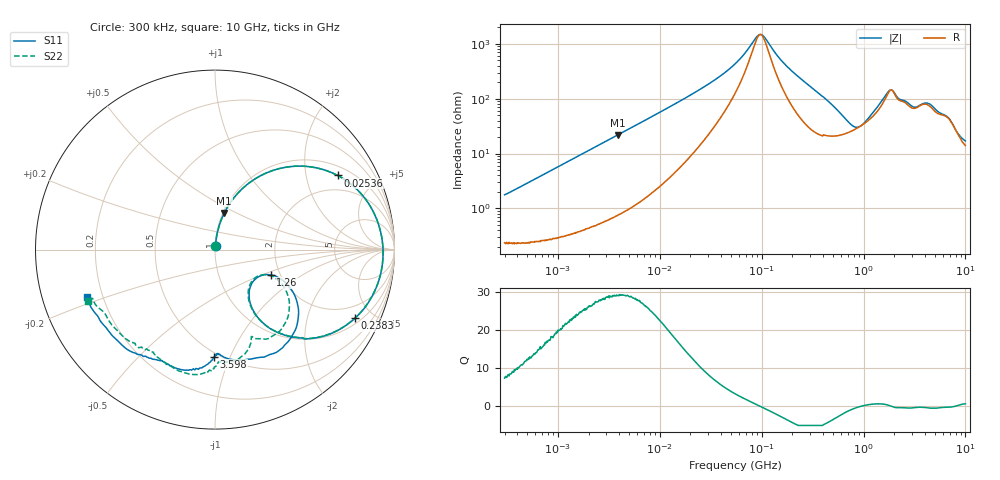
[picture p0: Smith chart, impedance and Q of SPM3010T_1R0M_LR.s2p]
! S-Parameter Data Generated by TDK Corporation
! Copyright(C) 2019 TDK Corporation.
! All Rights Reserved.
! TDK P/N: SPM3010T-1R0M-LR (Inductor)
! Property: L=1uH at 100kHz
! Size(LxWxT): 3.2x3x1mm
! Model Type: s2p (Touchstone File Format Version 1.0)
! Frequency: DC=Yes Start=0.3MHz Stop=10000MHz 802points Log-sweep
! Model Generated on Sep. 23, 2019
! Port Assignments:
!  1 ---@@@--- 2
! Applicable Conditions:
!  Temperature = 25 degC
!  DC Bias Current = 0 A
!  Small Signal Operation
! Terms and conditions regarding TDK Simulation Models
! (1)This simulation model is being provided solely for informational purposes. Please refer to the specifications of the products in terms of detailed characteristics of such products.
! (2)In no event shall TDK Corporation of any of its subsidiaries be liable for any loss or damage arising, directly or indirectly,
!  From any information contained in this simulation model, including, but not limited to loss or damages arising from any inaccuracies, omissions or errors in connection with such information.
! (3)Any and all copyrights on this simulation model are owned by TDK Corporation.
!  Duplication or redistribution of this simulation model without prior written permission from TDK Corporation is prohibited.
! (4)This simulation model is subject to any modification or change without any prior notice.
! (5)Neither TDK Corporation nor any of its subsidiaries shall make any warranty, express or implied,
!  Including but not limited to the correctness, implied warranties of merchantability and fitness for a particular purpose with respect to this simulation models.
! (6)The use of this simulation model shall be deemed to have consented to the terms and conditions hereof.
# Hz S MA R 50
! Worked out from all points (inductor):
!   801 points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, 300 kHz to 10 GHz, reference 50 ohm
!   read as one part in series: L = 916 nH near 318.3 kHz
!   highest Q = 29.1 at 3.867 MHz (marker M1), where L = 896 nH
!   self-resonance near 97.29 MHz
!   S11 on the Smith chart (normalised r, x): 300 kHz: 1.00, +0.04; 25.36 MHz: 1.34, +3.05; 238.3 MHz: 1.26, -3.94; 1.26 GHz: 1.79, -0.57; 3.598 GHz: 0.47, -0.87; 10 GHz: 0.14, -0.18
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300000  0.01837 81.3  0.9974 -1.0  0.9976 -0.9  0.0181 82.0
1713600  0.0964 82.1  0.9913 -5.5  0.9916 -5.5  0.09641 82.2
3866967  0.2107 75.8  0.9701 -12.2  0.9705 -12.2  0.2108 75.8
9671944  0.4691 59.3  0.8626 -28.1  0.8632 -28.1  0.469 59.3
2.53611e7  0.7983 31.2  0.5288 -53.2  0.5291 -53.2  0.7982 31.2
5.477226e7  0.9168 10.6  0.2138 -62.6  0.2139 -62.6  0.9167 10.6
9.914192e7  0.937 -2.6  0.06343 3.4  0.06346 3.4  0.9368 -2.6
1.473106e8  0.9261 -12.0  0.1629 55.5  0.163 55.4  0.9258 -11.9
2.382595e8  0.8692 -26.1  0.359 53.2  0.3591 53.2  0.8683 -26.1
3.126428e8  0.7984 -35.8  0.4859 44.8  0.4862 44.8  0.797 -35.9
4.687561e8  0.6178 -50.7  0.658 26.5  0.6583 26.5  0.615 -50.6
6.987102e8  0.3875 -57.7  0.7528 4.2  0.7532 4.1  0.382 -58.0
9.67469e8  0.277 -40.8  0.7342 -15.3  0.7345 -15.3  0.2704 -40.8
1.260284e9  0.3417 -24.4  0.6452 -31.6  0.6454 -31.6  0.3374 -25.3
1.525386e9  0.4646 -26.7  0.5179 -42.4  0.5181 -42.4  0.4567 -30.0
1.767019e9  0.5914 -38.2  0.3858 -42.0  0.386 -42.1  0.5598 -44.4
2.203374e9  0.6583 -65.4  0.4114 -27.9  0.4119 -27.9  0.5253 -67.2
2.756092e9  0.6149 -82.8  0.4284 -32.4  0.4286 -32.5  0.6176 -76.8
3.598403e9  0.5969 -90.5  0.408 -47.0  0.4082 -47.1  0.6366 -88.9
4.749267e9  0.6888 -103.0  0.365 -48.8  0.365 -48.8  0.7081 -101.3
6.899057e9  0.7157 -124.9  0.3501 -67.6  0.3501 -67.7  0.6789 -124.8
1e10  0.7612 -159.5  0.2995 -96.0  0.3 -96.3  0.7636 -157.9
